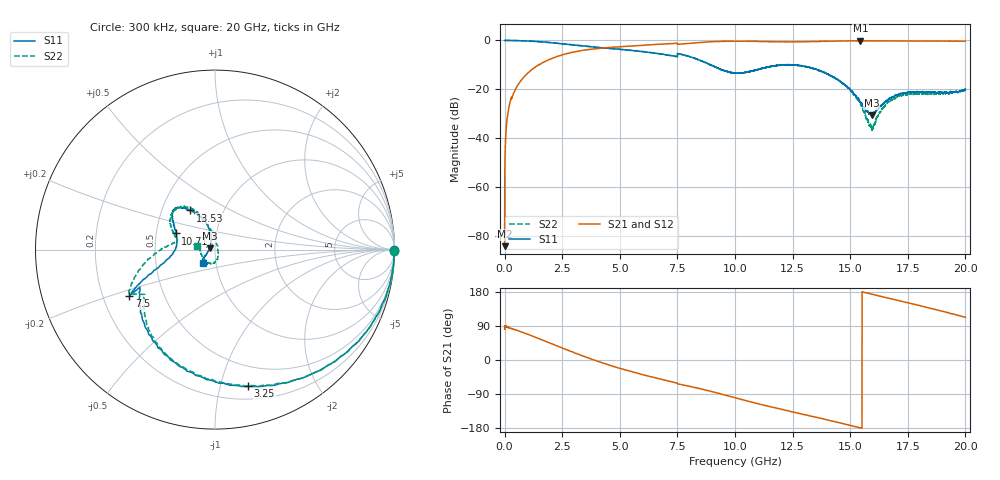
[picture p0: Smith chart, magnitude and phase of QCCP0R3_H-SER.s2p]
!{QCCP0R3}
!Johanson Technology Inc.
!www.johansontechnology.com
!Test Board Conditions:
!Substrate Type  RO4350B
!Substrate Thickness  20 mil
!Substrate Dk  3.66
!TL Type: GCPW
!TL Trace Width  36 mil
!TL Gap  12 mil
!Electrode orientation  Horizontal
!DUT TOPOLOGY	SERIES
!Mounting Pad LxW  26x36 mil
! Created Sat Jan  9 18:23:55 2021
# hz S ma R 50
! 2 Port Network Data from SP1.SP block
! freq  magS11  angS11  magS21  angS21  magS12  angS12  magS22  angS22
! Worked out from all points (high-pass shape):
!   20001 points, 300 kHz to 20 GHz, reference 50 ohm
!   highest |S21| = -0.13 dB at 15.44 GHz (marker M1); lowest = -84.0 dB at 300 kHz (marker M2)
!   |S21| within 3 dB of the highest: 4.241237 GHz to 4.241428 GHz (190.6 kHz wide, 0.00449 % of centre); 4.247 GHz to end of sweep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
!   lowest |S11| = -30.5 dB at 15.94 GHz (marker M3), VSWR 1.06, Z = 47.2 + j0.606 ohm
!   |S11| at or under -10 dB: 8.953 GHz to 11.97 GHz (3.012 GHz wide, 28.8 % of centre); 11.96559 GHz to 12.01527 GHz (49.68 MHz wide, 0.414 % of centre); 12.62 GHz to end of sweep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
!   |S22| runs from -36.8 to 0.0 dB; largest |S21 - S12| = 0.01
!   S11 on the Smith chart (normalised r, x): 300 kHz: open; 3.25 GHz: 0.31, -1.22; 7.5 GHz: 0.31, -0.23; 10.71 GHz: 0.63, +0.12; 13.53 GHz: 0.70, +0.33; 20 GHz: 0.87, -0.13
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300000  0.9948 -0.2  6.289e-05 80.8  0.0001304 115.8  0.9968 -0.3
1.023e8  0.9972 -2.4  0.02369 87.6  0.02373 87.4  0.9972 -2.3
1.363e8  0.9987 -3.2  0.0317 86.6  0.03163 86.6  0.9995 -3.2
2.623e8  0.9968 -6.1  0.06096 83.5  0.06091 83.4  0.998 -6.1
5.073e8  0.9937 -10.9  0.1082 78.7  0.108 78.7  0.9932 -10.9
1.4643e9  0.9462 -33.1  0.3157 56.8  0.3146 56.7  0.9483 -32.9
3.2503e9  0.7838 -76.4  0.6095 13.9  0.6098 14.0  0.7829 -75.3
3.3343e9  0.7784 -78.4  0.6217 12.0  0.6206 12.0  0.7798 -77.2
5.0273e9  0.6584 -112.5  0.7456 -22.4  0.7452 -22.3  0.6577 -111.4
6.6673e9  0.5402 -140.4  0.8343 -48.9  0.8353 -48.9  0.5377 -136.4
7.5003e9  0.5436 -151.5  0.8311 -62.8  0.8332 -62.9  0.5387 -152.8
1.00003e10  0.2185 176.2  0.965 -99.6  0.9657 -99.5  0.2181 167.0
1.07123e10  0.236 157.6  0.963 -110.9  0.9622 -111.0  0.2381 160.7
1.21413e10  0.3182 137.2  0.9376 -132.0  0.9378 -132.1  0.3126 139.2
1.33343e10  0.2737 124.0  0.9497 -148.5  0.9503 -148.7  0.2702 121.1
1.35343e10  0.2573 122.1  0.957 -151.6  0.956 -151.5  0.2556 118.1
1.46513e10  0.1351 106.5  0.9769 -167.5  0.9764 -167.4  0.1338 105.4
1.54393e10  0.05445 111.2  0.9853 -179.0  0.9815 -179.0  0.05067 87.5
1.59433e10  0.02977 167.6  0.9809 173.6  0.9799 173.6  0.01516 5.8
1.66673e10  0.06321 -149.1  0.9771 163.1  0.9773 163.0  0.05583 -74.9
1.75763e10  0.08742 -139.6  0.9767 149.8  0.9755 149.7  0.08151 -105.8
2e10  0.0981 -132.4  0.9674 112.7  0.9659 112.7  0.1019 168.1
